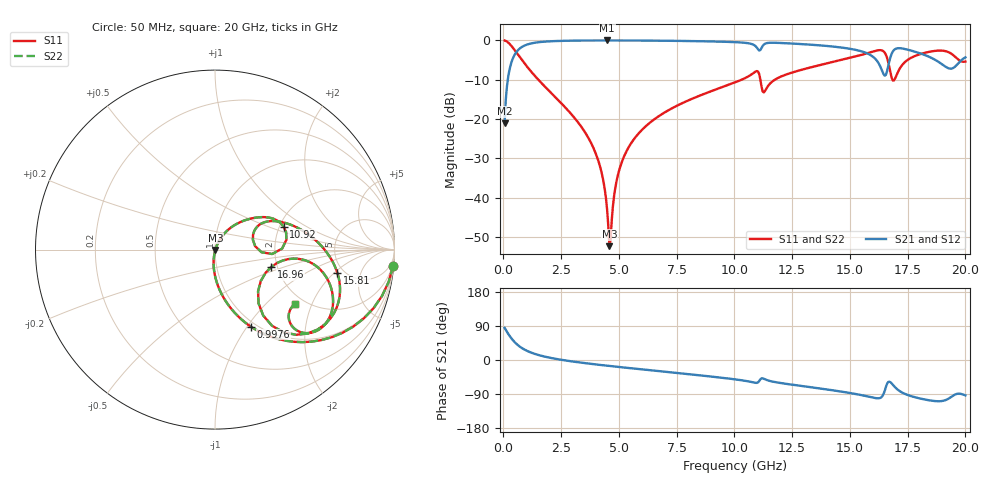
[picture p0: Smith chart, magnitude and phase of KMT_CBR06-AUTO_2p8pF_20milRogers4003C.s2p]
! Data measured by Modelithics Inc. support@modelithics.com 813-866-6335
! KEMET CBR06-AUTO 2.8pF, Pad Width= 0.851mm, Pad Length= 0.64mm, Pad Gap= 0.62mm, 20mil Rogers 4003C substrate Data, January 2022
# hz S ma R 50
! 2 Port Network Data from SP1.SP block
! freq  magS11  angS11  magS21  angS21  magS12  angS12  magS22  angS22
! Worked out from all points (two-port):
!   401 points, 50 MHz to 20 GHz, reference 50 ohm
!   highest |S21| = -0.02 dB at 4.489 GHz (marker M1); lowest = -21.0 dB at 50 MHz (marker M2)
!   |S21| within 3 dB of the highest: 553.7 MHz to 15.63 GHz (15.07 GHz wide, 186 % of centre); 16.84 GHz to 17.9 GHz (1.055 GHz wide, 6.07 % of centre)
!   lowest |S11| = -52.3 dB at 4.589 GHz (marker M3), VSWR 1.00, Z = 50.2 - j0.154 ohm
!   |S11| at or under -10 dB: 1.512 GHz to 10.31 GHz (8.798 GHz wide, 149 % of centre); 11.12 GHz to 11.75 GHz (622.9 MHz wide, 5.45 % of centre); 16.84323 GHz to 16.92444 GHz (81.21 MHz wide, 0.481 % of centre)
!   |S22| runs from -52.3 to 0.0 dB; largest |S21 - S12| = 0
!   S11 on the Smith chart (normalised r, x): 50 MHz: 1, -22; 997.6 MHz: 0.94, -1.04; 10.92 GHz: 2.10, +0.64; 15.81 GHz: 4.39, -2.20; 16.96 GHz: 1.86, -0.40; 20 GHz: 1.77, -1.52
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5e7  0.996 -5.3  0.08874 84.7  0.08874 84.7  0.996 -5.3
3.4925e8  0.8473 -33.2  0.5301 56.7  0.5301 56.7  0.8473 -33.2
9.97625e8  0.4733 -65.0  0.8796 24.8  0.8796 24.8  0.4733 -65.0
3.391625e9  0.07833 -95.8  0.9949 -7.2  0.9949 -7.2  0.07833 -95.8
4.13975e9  0.02758 -98.3  0.9974 -12.7  0.9974 -12.7  0.02758 -98.3
4.488875e9  0.007031 -86.8  0.9976 -15.1  0.9976 -15.1  0.007031 -86.8
4.588625e9  0.002432 -39.1  0.9976 -15.7  0.9976 -15.7  0.002432 -39.1
4.93775e9  0.01852 64.8  0.9973 -18.0  0.9973 -18.0  0.01852 64.8
5.237e9  0.03437 66.0  0.9968 -19.9  0.9968 -19.9  0.03437 66.0
6.73325e9  0.1093 59.2  0.9909 -29.3  0.9909 -29.3  0.1093 59.2
1.0025e10  0.2923 37.7  0.9494 -51.1  0.9494 -51.1  0.2923 37.7
1.092275e10  0.403 18.5  0.8401 -60.3  0.8401 -60.3  0.403 18.5
1.132175e10  0.2272 21.2  0.9057 -50.8  0.9057 -50.8  0.2272 21.2
1.336662e10  0.459 16.6  0.8792 -72.3  0.8792 -72.3  0.459 16.6
1.58105e10  0.6942 -10.8  0.6705 -96.7  0.6705 -96.7  0.6942 -10.8
1.630925e10  0.7517 -27.7  0.4699 -100.2  0.4699 -100.2  0.7517 -27.7
1.650875e10  0.697 -42.1  0.3559 -80.9  0.3559 -80.9  0.697 -42.1
1.670825e10  0.4545 -53.8  0.5454 -57.2  0.5454 -57.2  0.4545 -53.8
1.695762e10  0.3285 -17.0  0.7743 -72.1  0.7743 -72.1  0.3285 -17.0
1.825438e10  0.6964 -20.2  0.6498 -104.4  0.6498 -104.4  0.6964 -20.2
1.930175e10  0.7011 -41.5  0.4393 -100.9  0.4393 -100.9  0.7011 -41.5
2e10  0.5385 -34.4  0.609 -93.4  0.609 -93.4  0.5385 -34.4
